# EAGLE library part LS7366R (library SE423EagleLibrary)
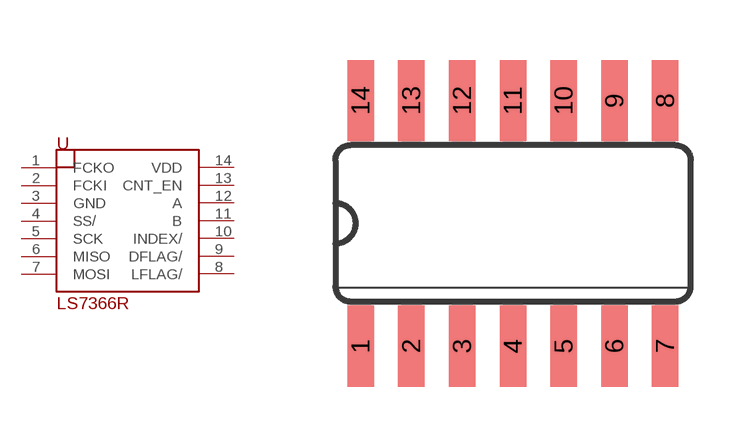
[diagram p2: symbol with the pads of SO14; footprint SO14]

Designator prefix U

## LS7366R  [SO14]
1  FCKO
2  FCKI
3  GND
4  SS/
5  SCK
6  MISO
7  MOSI
8  LFLAG/
9  DFLAG/
10  INDEX/
11  B
12  A
13  CNT_EN
14  VDD

## Footprint SO14 (pad centres in mm)
Small Outline package 150 mil
smd 0.66 x 2.032: 1 -3.81,-3.073; 2 -2.54,-3.073; 3 -1.27,-3.073; 4 0,-3.073; 5 1.27,-3.073; 6 2.54,-3.073; 7 3.81,-3.073; 8 3.81,3.073; 9 2.54,3.073; 10 1.27,3.073; 11 0,3.073; 12 -1.27,3.073; 13 -2.54,3.073; 14 -3.81,3.073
